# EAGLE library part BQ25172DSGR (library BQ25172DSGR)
Battery Management 0.8-A, one- to six-cell NiMH stand-alone linear charger in a QFN package Source: Datasheet
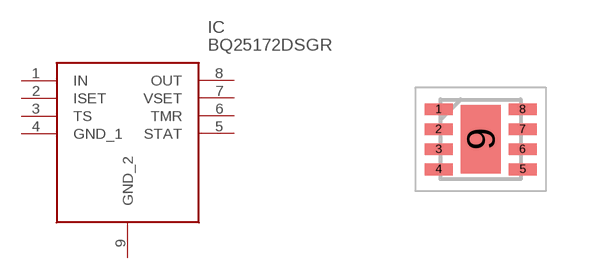
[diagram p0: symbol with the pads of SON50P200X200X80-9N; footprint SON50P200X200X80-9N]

Designator prefix IC

## BQ25172DSGR (Description: Battery Management 0.8-A, one- to six-cell NiMH stand-alone linear charger in a QFN package; Height: 0.8mm; Manufacturer_Name: Texas Instruments; Manufacturer_Part_Number: BQ25172DSGR; Mouser_Part_Number: 595-BQ25172DSGR; Mouser_Price-Stock: https://www.mouser.co.uk/ProductDetail/Texas-Instruments/BQ25172DSGR?qs=tlsG%2FOw5FFgckLJXIVn4PA%3D%3D)  [SON50P200X200X80-9N]
1  IN
2  ISET
3  TS
4  GND_1
5  STAT
6  TMR
7  VSET
8  OUT
9  GND_2

## Footprint SON50P200X200X80-9N (pad centres in mm)
DSG0008A _ 2021
smd 0.7 x 0.3: 1 -1.05,0.75; 2 -1.05,0.25; 3 -1.05,-0.25; 4 -1.05,-0.75; 5 1.05,-0.75; 6 1.05,-0.25; 7 1.05,0.25; 8 1.05,0.75
smd 1 x 1.7: 9 0,0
